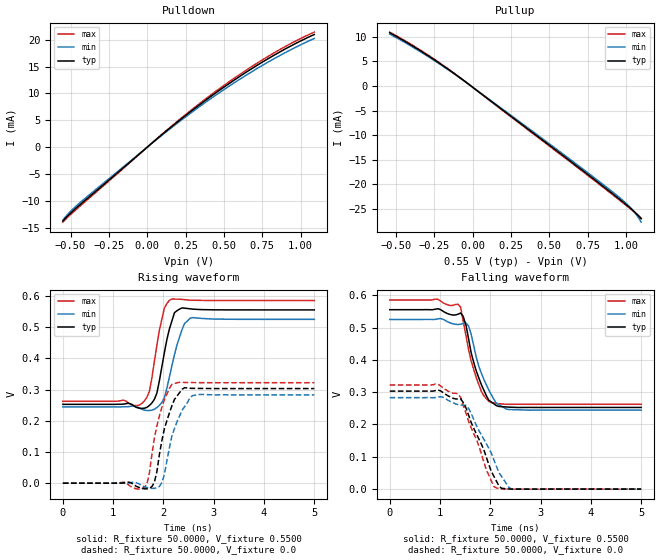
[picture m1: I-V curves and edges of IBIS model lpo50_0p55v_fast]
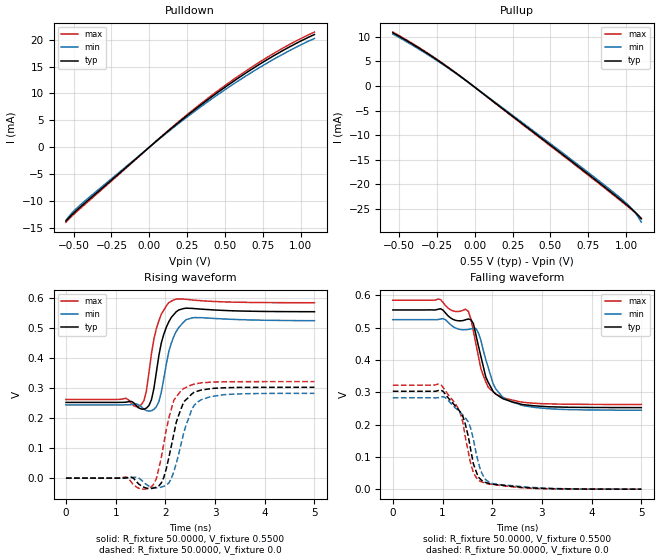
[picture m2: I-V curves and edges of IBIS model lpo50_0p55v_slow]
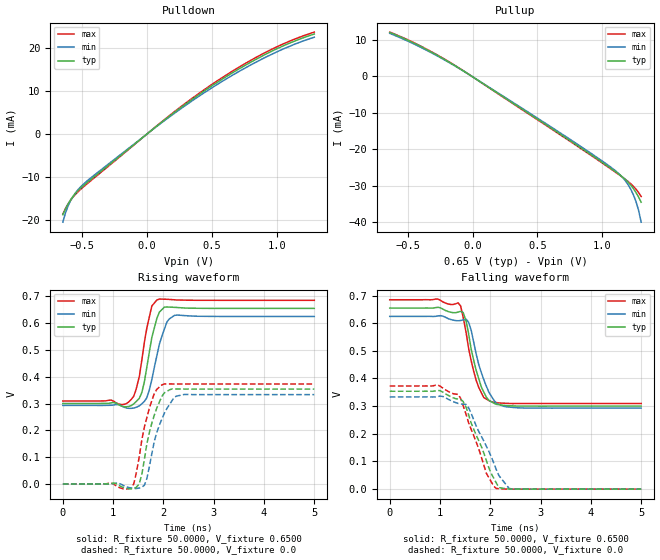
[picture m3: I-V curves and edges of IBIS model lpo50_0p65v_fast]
| Integrated Devices Technolgy, Inc
[Ibis Ver]   4.1
[File Name]   9dbl0941.ibs
[File Rev]   1.2
[Date]   5/4/2016
[Source]   Integrated Devices Technolgy, Inc.
[Notes]   Rev 1.0 created by sg ; 03/01/2016
   Rev 1.1 replace all LP-HCSL with rcx models ; 04/22/2016
   Rev 1.2 created additional DIFIN model; EvK, 05/04/2016
[Disclaimer] Integrated Device Technology, Inc. ("IDT") hereby grants the
   user of this IBIS model a non-exclusive, nontransferable
   license to use this IBIS model under the following terms. The
   user is granted this license only to use the IBIS model and is
   not granted rights to sell, copy (except as needed to run the
   IBIS model), rent, lease or sub-license the IBIS model in
   whole or in part, or in modified form to anyone. The User may
   modify the IBIS model to suit its specific applications, but
   rights to derivative works and such modifications shall belong
   to IDT. This IBIS model is provided on an AS IS" basis and IDT
   makes absolutely no warranty with respect to the information
   contained herein. IDT DISCLAIMS AND CUSTOMER WAIVES ALL
   WARRANTIES, EXPRESS AND IMPLIED, INCLUDING WARRANTIES OF
   MERCHANTABILITY AND FITNESS FOR A PARTICULAR PURPOSE. THE
   ENTIRE RISK AS TO QUALITY AND PERFORMANCE IS WITH THE USER
   ACCORDINGLY, IN NO EVENT SHALL IDT BE LIABLE FOR ANY DIRECT OR
   INDIRECT DAMAGES, WHETHER IN CONTRACT OR TORT, INCLUDING ANY
   LOST PROFITS OR OTHER INCIDENTAL, CONSEQUENTIAL, EXEMPLARY, OR
   PUNITIVE DAMAGES ARISING OUT OF THE USE OR APPLICATION OF THE
   IBIS model. Further, IDT reserves the right to make changes
   without notice to any product herein to improve reliability,
   function, or design. IDT does not convey any license under
   patent rights or any other intellectual property rights,
   including those of third parties. IDT is not obligated to
   provide maintenance or support for the licensed IBIS model.
[Copyright]   Copyright 2006, Integrated Devices Technolgy, Inc. all rights
   reserved
|   COMPONENT: 9dbl0941
[Component]   IDT9dbl0941
[Manufacturer]   Integrated Device Technology, Inc.
[Package]
| variable   typ   min   max
R_pkg   72.4655m   58.8860m   86.0450m
L_pkg   1.4717nH   1.1165nH   1.7785nH
C_pkg   77.4700fF   74.4400fF   80.5000fF
[Pin]  signal_name   model_name   R_pin   L_pin   C_pin
1   vSADR_tri   IN
2   vOE8#   IN
3   DIF8   LPO
4   DIF8#   LPO
5   VDDR3.3   POWER
6   CLK_IN   DIFIN
7   CLK_IN#   DIFIN
8   GNDR   GND
9   GNDDIG   GND
10   SCL_3.3   SCL
11   SDATA_3.3   SDA
12   VDDDIG3.3   POWER
13   VDDIO   POWER
14   vOE0#   IN
15   DIF0   LPO
16   DIF0#   LPO
17   vOE1#   IN
18   DIF1   LPO
19   DIF1#   LPO
20   VDD3.3   POWER
21   VDDIO   POWER
22   GND   GND
23   DIF2   LPO
24   DIF2#   LPO
25   vOE2#   IN
26   DIF3   LPO
27   DIF3#   LPO
28   vOE3#   IN
29   GNDA   GND
30   VDDA3.3   POWER
31   VDDIO   POWER
32   DIF4   LPO
33   DIF4#   LPO
34   vOE4#   IN
35   DIF5   LPO
36   DIF5#   LPO
37   vOE5#   IN
38   VDD3.3   POWER
39   VDDIO   POWER
40   GND   GND
41   DIF6   LPO
42   DIF6#   LPO
43   vOE6#   IN
44   DIF7   LPO
45   DIF7#   LPO
46   vOE7#   IN
47   VDDIO   POWER
48   CLKPWRGD_PD#   IN
49   EPAD   GND
[Diff Pin]   inv_pin   vdiff   tdelay_typ   tdelay_min   tdelay_max
3   4   NA   NA
6   7   NA   NA
15   16   NA   NA
18   19   NA   NA
23   24   NA   NA
26   27   NA   NA
29   30   NA   NA
32   33   NA   NA
35   36   NA   NA
41   42   NA   NA
44   45   NA   NA
[Model Selector] LPO
lpo50_0p55v_fast amplitude 0.55V, slew rate fast
lpo50_0p55v_slow amplitude 0.55V, slew rate slow
lpo50_0p65v_fast amplitude 0.65V, slew rate fast
lpo50_0p65v_slow amplitude 0.65V, slew rate slow
lpo50_0p7v_fast amplitude 0.7V, slew rate fast
lpo50_0p7v_slow amplitude 0.7V, slew rate slow
lpo50_0p8v_fast amplitude 0.8V, slew rate fast
lpo50_0p8v_slow amplitude 0.8V, slew rate slow
| Models and submodels in the file (12): lpo50_0p55v_fast (Output), lpo50_0p55v_slow (Output), lpo50_0p65v_fast (Output), lpo50_0p65v_slow (Output), lpo50_0p7v_fast (Output), lpo50_0p7v_slow (Output), lpo50_0p8v_fast (Output), lpo50_0p8v_slow (Output), SDA (I/O_open_drain), SCL (Input), IN (Input), DIFIN (Input)
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|   Model lpo50_0p55v_fast
[Model]  lpo50_0p55v_fast
Model_type Output
Polarity   Non-Inverting
Vmeas =  0.4000V
Cref =   2.0000pF
Rref =   0.0
Vref =   0.4000V
C_comp   1.1000pF   1.0000pF   1.2000pF
[Temperature Range]   27.0000   70.0000   0.0
[Voltage Range]   0.5500V   0.5200V   0.5800V
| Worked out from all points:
|   slope of the pulldown table from 0 to 0.083 V, typ, clamps not added: 41.1 ohm
|   slope of the pullup table from 0 to 0.083 V, typ, clamps not added: 42.2 ohm
|   rising waveform, R_fixture 50.0000, V_fixture 0.5500: 20-80 % time 219ps typ, 260ps min, 204ps max; typ from 0.253 V to 0.555 V
|   rising waveform, R_fixture 50.0000, V_fixture 0.0: 20-80 % time 265ps typ, 299ps min, 252ps max; typ from 0 V to 0.303 V
|   falling waveform, R_fixture 50.0000, V_fixture 0.5500: 20-80 % time 319ps typ, 357ps min, 304ps max; typ from 0.555 V to 0.253 V
|   falling waveform, R_fixture 50.0000, V_fixture 0.0: 20-80 % time 469ps typ, 516ps min, 447ps max; typ from 0.303 V to 0 V
[Pulldown]
|Voltage   I(typ)   I(min)   I(max)
-550mV    -13.73mA   -13.58mA   -13.94mA
-490mV    -11.99mA   -11.64mA   -12.27mA
-370mV    -9.029mA   -8.682mA   -9.273mA
130mV     3.135mA    2.995mA    3.234mA
390mV     8.917mA    8.541mA    9.18mA
590mV     12.91mA    12.39mA    13.27mA
770mV     16.15mA    15.52mA    16.57mA
930mV     18.72mA    18.03mA    19.18mA
1.09V     20.96mA    20.22mA    21.41mA
[Pullup]
|Voltage   I(typ)   I(min)   I(max)
-540mV    10.83mA    10.57mA    10.97mA
-360mV    7.564mA    7.356mA    7.689mA
-160mV    3.433mA    3.328mA    3.503mA
580mV     -13.9mA    -13.59mA   -14.09mA
840mV     -20.11mA   -19.75mA   -20.32mA
980mV     -23.56mA   -23.25mA   -23.75mA
1.04V     -25.13mA   -25.06mA   -25.26mA
1.08V     -26.32mA   -26.68mA   -26.31mA
1.1V      -27.01mA   -27.7mA    -26.88mA
[Ramp]
| variable   typ   min   max
dV/dt_r  0.1819/0.2649n   0.1698/0.2989n   0.1933/0.2519n
dV/dt_f  0.1815/0.3187n   0.1683/0.3570n   0.1937/0.2938n
R_load = 50.0000
[Rising Waveform]
R_fixture= 50.0000
V_fixture= 0.5500
V_fixture_min= 0.5200
V_fixture_max= 0.5800
|time   V(typ)   V(min)   V(max)
0s        252.7mV    244.5mV    262.4mV
1.57ns    239.7mV    236.8mV    255.1mV
1.72ns    248.9mV    232.8mV    294.2mV
1.87ns    288.9mV    242.3mV    442.4mV
2.02ns    419.2mV    274.6mV    561.9mV
2.17ns    520.6mV    377.6mV    590mV
2.22ns    546.4mV    411.6mV    589.9mV
2.37ns    561.6mV    492.2mV    589mV
2.53ns    558.7mV    528.5mV    586.4mV
5ns       555.2mV    525mV      585.3mV
[Rising Waveform]
R_fixture= 50.0000
V_fixture= 0.0
V_fixture_min= 0.0
V_fixture_max= 0.0
|time   V(typ)   V(min)   V(max)
0s        1.148uV    712.2nV    1.484uV
1.31ns    3.407mV    809.2uV    -6.162mV
1.62ns    -17.94mV   -11.39mV   -13.71mV
1.72ns    -15.85mV   -15.73mV   31.64mV
1.82ns    3.269mV    -16.45mV   144.5mV
1.97ns    137.4mV    2.416mV    243.4mV
2.17ns    248.9mV    152.2mV    316.8mV
2.37ns    300.7mV    233.4mV    323.1mV
2.58ns    303.8mV    280.8mV    322.4mV
5ns       303.2mV    283mV      322.1mV
[Falling Waveform]
R_fixture= 50.0000
V_fixture= 0.5500
V_fixture_min= 0.5200
V_fixture_max= 0.5800
|time   V(typ)   V(min)   V(max)
0s        555.2mV    525mV      585.3mV
1.36ns    541.3mV    509.4mV    571.9mV
1.41ns    544.9mV    510.3mV    562.9mV
1.46ns    535mV      512.6mV    520.2mV
1.57ns    463.4mV    504.3mV    429.6mV
1.67ns    392.3mV    443.4mV    370.2mV
1.82ns    323.8mV    359.3mV    303mV
2.02ns    269.5mV    292.3mV    268.1mV
2.37ns    253.6mV    246.2mV    262.4mV
5ns       252.7mV    244.5mV    262.4mV
[Falling Waveform]
R_fixture= 50.0000
V_fixture= 0.0
V_fixture_min= 0.0
V_fixture_max= 0.0
|time   V(typ)   V(min)   V(max)
0s        303.2mV    283mV      322.1mV
960ps     306.4mV    284.8mV    324.5mV
1.36ns    278.7mV    261.3mV    294mV
1.46ns    268.3mV    260.1mV    259.6mV
1.57ns    227.9mV    249.2mV    209.7mV
1.92ns    99.15mV    140.5mV    60.22mV
2.12ns    25.15mV    70.99mV    3.548mV
2.22ns    2.568mV    39.83mV    933.4uV
2.42ns    88.16uV    302.9uV    -182.1uV
5ns       1.862uV    1.201uV    2.782uV
|   Model lpo50_0p55v_slow
[Model]  lpo50_0p55v_slow
Model_type Output
Polarity   Non-Inverting
Vmeas =  0.4000V
Cref =   2.0000pF
Rref =   0.0
Vref =   0.4000V
C_comp   1.1000pF   1.0000pF   1.2000pF
[Temperature Range]   27.0000   70.0000   0.0
[Voltage Range]   0.5500V   0.5200V   0.5800V
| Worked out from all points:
|   slope of the pulldown table from 0 to 0.083 V, typ, clamps not added: 41.1 ohm
|   slope of the pullup table from 0 to 0.083 V, typ, clamps not added: 42.2 ohm
|   rising waveform, R_fixture 50.0000, V_fixture 0.5500: 20-80 % time 218ps typ, 228ps min, 213ps max; typ from 0.253 V to 0.555 V
|   rising waveform, R_fixture 50.0000, V_fixture 0.0: 20-80 % time 283ps typ, 294ps min, 254ps max; typ from 0 V to 0.303 V
|   falling waveform, R_fixture 50.0000, V_fixture 0.5500: 20-80 % time 334ps typ, 371ps min, 308ps max; typ from 0.555 V to 0.253 V
|   falling waveform, R_fixture 50.0000, V_fixture 0.0: 20-80 % time 322ps typ, 344ps min, 308ps max; typ from 0.303 V to 0 V
[Pulldown]
|Voltage   I(typ)   I(min)   I(max)
-550mV    -13.73mA   -13.58mA   -13.94mA
-490mV    -11.99mA   -11.64mA   -12.27mA
-370mV    -9.029mA   -8.682mA   -9.273mA
130mV     3.135mA    2.995mA    3.234mA
390mV     8.917mA    8.541mA    9.18mA
590mV     12.91mA    12.39mA    13.27mA
770mV     16.15mA    15.52mA    16.57mA
930mV     18.72mA    18.03mA    19.18mA
1.09V     20.96mA    20.22mA    21.41mA
[Pullup]
|Voltage   I(typ)   I(min)   I(max)
-540mV    10.83mA    10.57mA    10.97mA
-360mV    7.564mA    7.356mA    7.689mA
-160mV    3.433mA    3.328mA    3.503mA
580mV     -13.9mA    -13.59mA   -14.09mA
840mV     -20.11mA   -19.75mA   -20.32mA
980mV     -23.56mA   -23.25mA   -23.75mA
1.04V     -25.13mA   -25.06mA   -25.26mA
1.08V     -26.32mA   -26.68mA   -26.31mA
1.1V      -27.01mA   -27.7mA    -26.88mA
[Ramp]
| variable   typ   min   max
dV/dt_r  0.1819/0.2830n   0.1697/0.3065n   0.1933/0.2544n
dV/dt_f  0.1815/0.3340n   0.1682/0.3711n   0.1937/0.3078n
R_load = 50.0000
[Rising Waveform]
R_fixture= 50.0000
V_fixture= 0.5500
V_fixture_min= 0.5200
V_fixture_max= 0.5800
|time   V(typ)   V(min)   V(max)
0s        252.7mV    244.5mV    262.4mV
1.31ns    256.4mV    245.3mV    250.3mV
1.52ns    230.5mV    237.8mV    245.9mV
1.62ns    233.9mV    225.4mV    292.8mV
1.72ns    261.4mV    224.9mV    414.6mV
1.87ns    409.5mV    255.5mV    524.9mV
2.02ns    503.8mV    381mV      574.6mV
2.17ns    545.9mV    472.6mV    594.8mV
2.58ns    565.8mV    535.9mV    593.8mV
5ns       555.4mV    525.4mV    585.4mV
[Rising Waveform]
R_fixture= 50.0000
V_fixture= 0.0
V_fixture_min= 0.0
V_fixture_max= 0.0
|time   V(typ)   V(min)   V(max)
0s        1.148uV    712.1nV    1.484uV
1.31ns    3.844mV    793.7uV    -12.27mV
1.72ns    -34.68mV   -29.54mV   -29.1mV
1.82ns    -30.19mV   -32.36mV   -1.057mV
1.97ns    2.981mV    -27.23mV   116.9mV
2.17ns    146.9mV    21mV       259.8mV
2.37ns    254.6mV    151.2mV    299mV
2.53ns    280.7mV    228.5mV    311.2mV
3.13ns    301.1mV    277.4mV    321.3mV
5ns       303.2mV    282.9mV    322.1mV
[Falling Waveform]
R_fixture= 50.0000
V_fixture= 0.5500
V_fixture_min= 0.5200
V_fixture_max= 0.5800
|time   V(typ)   V(min)   V(max)
0s        555.2mV    525mV      585.3mV
910ps     557.3mV    525.4mV    588.9mV
1.52ns    527.3mV    494.8mV    550.6mV
1.67ns    479.6mV    498.1mV    451.7mV
1.77ns    412.5mV    461.9mV    374.3mV
1.87ns    347.7mV    401.7mV    333.1mV
2.02ns    302.3mV    325.9mV    301.3mV
2.22ns    279.9mV    283.2mV    284.1mV
2.93ns    257.3mV    252mV      265.4mV
5ns       252.7mV    244.6mV    262.5mV
[Falling Waveform]
R_fixture= 50.0000
V_fixture= 0.0
V_fixture_min= 0.0
V_fixture_max= 0.0
|time   V(typ)   V(min)   V(max)
0s        303.2mV    283mV      322.1mV
960ps     307.1mV    285.3mV    324.6mV
1.36ns    238.6mV    237.1mV    234.4mV
1.41ns    225.1mV    229.5mV    206.5mV
1.52ns    162.1mV    208.1mV    114.1mV
1.62ns    79.19mV    154.8mV    51.67mV
1.77ns    30.02mV    57.01mV    23.61mV
1.87ns    20.45mV    28.85mV    17.79mV
2.17ns    12.71mV    13.81mV    11.47mV
5ns       18.83uV    54.19uV    8.424uV
|   Model lpo50_0p65v_fast
[Model]  lpo50_0p65v_fast
Model_type Output
Polarity   Non-Inverting
Vmeas =  0.4000V
Cref =   2.0000pF
Rref =   0.0
Vref =   0.4000V
C_comp   1.1000pF   1.0000pF   1.2000pF
[Temperature Range]   27.0000   70.0000   0.0
[Voltage Range]   0.6500V   0.6200V   0.6800V
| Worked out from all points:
|   slope of the pulldown table from 0 to 0.098 V, typ, clamps not added: 41.2 ohm
|   slope of the pullup table from 0 to 0.098 V, typ, clamps not added: 43 ohm
|   rising waveform, R_fixture 50.0000, V_fixture 0.6500: 20-80 % time 213ps typ, 252ps min, 205ps max; typ from 0.3 V to 0.655 V
|   rising waveform, R_fixture 50.0000, V_fixture 0.0: 20-80 % time 265ps typ, 303ps min, 254ps max; typ from 0 V to 0.354 V
|   falling waveform, R_fixture 50.0000, V_fixture 0.6500: 20-80 % time 273ps typ, 312ps min, 264ps max; typ from 0.655 V to 0.3 V
|   falling waveform, R_fixture 50.0000, V_fixture 0.0: 20-80 % time 443ps typ, 492ps min, 426ps max; typ from 0.354 V to 0 V
[Pulldown]
|Voltage   I(typ)   I(min)   I(max)
-650mV    -18.76mA   -20.5mA    -18.62mA
-630mV    -17.42mA   -18.38mA   -17.37mA
-610mV    -16.28mA   -16.76mA   -16.29mA
-590mV    -15.29mA   -15.48mA   -15.38mA
-550mV    -13.73mA   -13.58mA   -13.94mA
-510mV    -12.53mA   -12.21mA   -12.79mA
-390mV    -9.514mA   -9.154mA   -9.768mA
170mV     4.068mA    3.887mA    4.195mA
470mV     10.56mA    10.12mA    10.87mA
770mV     16.15mA    15.52mA    16.57mA
1.03V     20.16mA    19.44mA    20.62mA
1.29V     23.19mA    22.45mA    23.64mA
[Pullup]
|Voltage   I(typ)   I(min)   I(max)
-640mV    11.97mA    11.72mA    12.07mA
-400mV    8.099mA    7.887mA    8.218mA
-140mV    2.942mA    2.851mA    3.002mA
660mV     -15.52mA   -15.2mA    -15.71mA
1.08V     -25.64mA   -25.34mA   -25.8mA
1.16V     -27.78mA   -27.91mA   -27.83mA
1.2V      -29.1mA    -29.81mA   -28.92mA
1.22V     -29.9mA    -31.04mA   -29.53mA
1.24V     -30.83mA   -32.53mA   -30.21mA
1.26V     -31.91mA   -34.39mA   -31mA
1.28V     -33.14mA   -36.79mA   -31.92mA
1.3V      -34.56mA   -40.04mA   -32.99mA
[Ramp]
| variable   typ   min   max
dV/dt_r  0.2123/0.2653n   0.2000/0.3029n   0.2237/0.2495n
dV/dt_f  0.2128/0.2733n   0.1990/0.3123n   0.2252/0.2560n
R_load = 50.0000
[Rising Waveform]
R_fixture= 50.0000
V_fixture= 0.6500
V_fixture_min= 0.6200
V_fixture_max= 0.6800
|time   V(typ)   V(min)   V(max)
0s        300.2mV    293mV      309.4mV
1.36ns    292.3mV    282.1mV    315.6mV
1.46ns    307.9mV    286.1mV    354.9mV
1.57ns    341mV      299mV      461.7mV
1.67ns    435.8mV    321.9mV    581.7mV
1.77ns    547mV      389.7mV    663.9mV
1.87ns    617.8mV    479mV      686mV
2.07ns    660mV      604.6mV    688.7mV
2.22ns    658.6mV    628.6mV    686.7mV
5ns       654.8mV    624.6mV    684.8mV
[Rising Waveform]
R_fixture= 50.0000
V_fixture= 0.0
V_fixture_min= 0.0
V_fixture_max= 0.0
|time   V(typ)   V(min)   V(max)
0s        731.2nV    0V         944.7nV
1.36ns    -18.23mV   -15.1mV    -13.61mV
1.41ns    -16.22mV   -16.62mV   430.6uV
1.52ns    1.282mV    -15.09mV   102.2mV
1.62ns    90.24mV    -4.963mV   211.4mV
1.82ns    257.5mV    160.6mV    337.6mV
1.97ns    327.1mV    242.4mV    369.5mV
2.22ns    354.4mV    324.5mV    373mV
2.42ns    354mV      334mV      373mV
5ns       353.9mV    333.3mV    372.9mV
[Falling Waveform]
R_fixture= 50.0000
V_fixture= 0.6500
V_fixture_min= 0.6200
V_fixture_max= 0.6800
|time   V(typ)   V(min)   V(max)
0s        654.8mV    624.6mV    684.8mV
1.36ns    640.1mV    608.8mV    673.6mV
1.46ns    638.6mV    611.9mV    622.5mV
1.57ns    560.5mV    602.9mV    507.2mV
1.72ns    428.7mV    487.9mV    393.2mV
1.87ns    350.6mV    396mV      330.9mV
2.02ns    316mV      336.3mV    316mV
2.12ns    306.6mV    310.6mV    313mV
2.53ns    300.3mV    294.1mV    309.4mV
5ns       300.2mV    293mV      309.4mV
[Falling Waveform]
R_fixture= 50.0000
V_fixture= 0.0
V_fixture_min= 0.0
V_fixture_max= 0.0
|time   V(typ)   V(min)   V(max)
0s        353.9mV    333.3mV    372.9mV
960ps     357.1mV    335.1mV    375.8mV
1.36ns    325.6mV    309.7mV    342.5mV
1.46ns    316.7mV    306.9mV    301.6mV
1.57ns    268mV      293.3mV    239mV
1.92ns    104.2mV    155.6mV    57.66mV
2.12ns    22.08mV    70.18mV    2.086mV
2.17ns    5.361mV    49.24mV    1.512mV
2.42ns    212uV      272.4uV    -43.07uV
5ns       1.896uV    857.7nV    1.146uV
